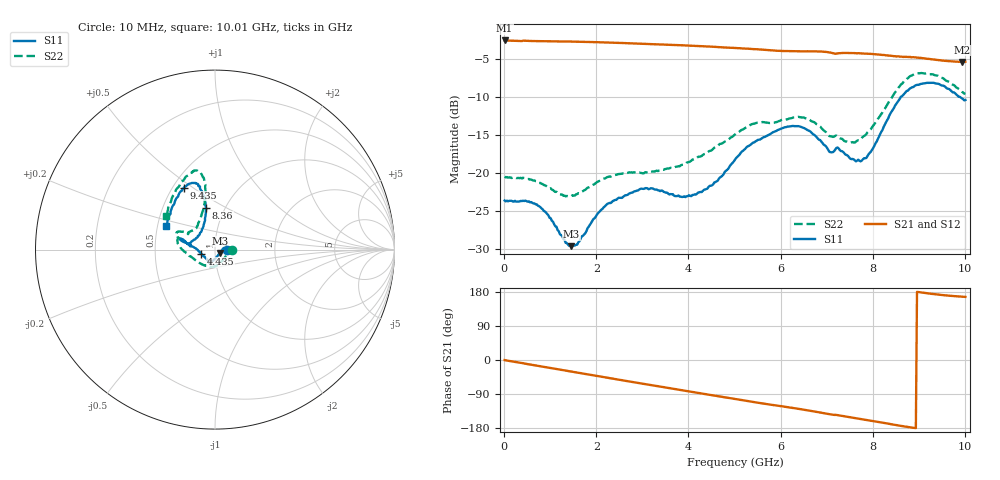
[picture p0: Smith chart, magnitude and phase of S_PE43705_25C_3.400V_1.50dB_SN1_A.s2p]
! Device ID: PE43705
! Serial: 1
! Insertion: A
! Impedance: 50 ohm
! Temp: 25C
! VDD: 3.400V
! Attenuation Step: 1.50dB
#  Hz  S  RI  R  50
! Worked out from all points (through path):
!   401 points, 10 MHz to 10.01 GHz, reference 50 ohm
!   highest |S21| = -2.52 dB at 10 MHz (marker M1); lowest = -5.4 dB at 9.935 GHz (marker M2)
!   group delay of S21, straight-line fit = 55 ps
!   lowest |S11| = -29.7 dB at 1.46 GHz (marker M3), VSWR 1.07, Z = 52.7 - j2 ohm
!   |S11| at or under -10 dB: start of sweep to 8.606 GHz; 9.897 GHz to end of sweep
!   |S22| runs from -23.1 to -6.8 dB; largest |S21 - S12| = 0.0069
!   S11 on the Smith chart (normalised r, x): 10 MHz: 1.14, -0.00; 4.435 GHz: 0.86, -0.04; 8.36 GHz: 0.81, +0.40; 9.435 GHz: 0.57, +0.46; 10.01 GHz: 0.55, +0.16
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1e7  0.0657 -0.000507  0.7479 -0.00361  0.7481 -0.0035  0.0945 -0.000606
7.35e8  0.0582 0.0171  0.7137 -0.1976  0.714 -0.1971  0.0864 0.00257
1.46e9  0.0268 -0.019  0.6329 -0.3739  0.6331 -0.374  0.053 -0.0459
1.685e9  0.0151 -0.035  0.5982 -0.4231  0.5982 -0.4234  0.0378 -0.0648
2.235e9  -0.0105 -0.0614  0.497 -0.5276  0.4974 -0.5272  -0.00112 -0.0937
2.96e9  -0.0305 -0.0723  0.3379 -0.6259  0.3384 -0.6254  -0.039 -0.0922
3.36e9  -0.0344 -0.0685  0.2452 -0.6597  0.2459 -0.6591  -0.0518 -0.0895
3.885e9  -0.0481 -0.0501  0.117 -0.6844  0.118 -0.6839  -0.0846 -0.0753
4.435e9  -0.0774 -0.023  -0.0171 -0.6825  -0.0157 -0.6818  -0.1319 -0.0414
5.01e9  -0.1214 0.0153  -0.1489 -0.6499  -0.1482 -0.6502  -0.1791 -0.00281
5.41e9  -0.1552 0.0327  -0.2321 -0.6134  -0.2314 -0.6139  -0.2078 0.0361
6.06e9  -0.1886 0.0611  -0.3444 -0.5361  -0.3426 -0.5361  -0.211 0.0771
6.685e9  -0.1768 0.0435  -0.447 -0.4492  -0.4472 -0.4485  -0.1933 0.1013
7.085e9  -0.1344 0.0256  -0.5002 -0.37  -0.5008 -0.3707  -0.151 0.0877
7.26e9  -0.1406 0.0348  -0.5098 -0.3459  -0.5082 -0.3471  -0.1386 0.1004
7.71e9  -0.0919 0.0777  -0.5588 -0.2577  -0.5576 -0.2592  -0.0979 0.1321
7.985e9  -0.0663 0.1257  -0.5759 -0.1991  -0.5748 -0.2028  -0.0775 0.1847
8.36e9  -0.0508 0.2336  -0.5825 -0.1179  -0.5814 -0.1212  -0.0546 0.2929
8.86e9  -0.0936 0.3558  -0.5798 -0.0152  -0.5757 -0.0185  -0.09 0.4319
9.435e9  -0.1741 0.3449  -0.5496 0.0722  -0.5482 0.0723  -0.1676 0.399
9.935e9  -0.2639 0.1638  -0.5265 0.12  -0.5289 0.1201  -0.262 0.2212
1.001e10  -0.2736 0.1295  -0.5268 0.1265  -0.5296 0.1251  -0.2737 0.1886
